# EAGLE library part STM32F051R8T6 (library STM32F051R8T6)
Entry-level ARM Cortex-M0 Access line MCU with 64 Kbytes Flash, 48 MHz CPU, motor control and CEC functions
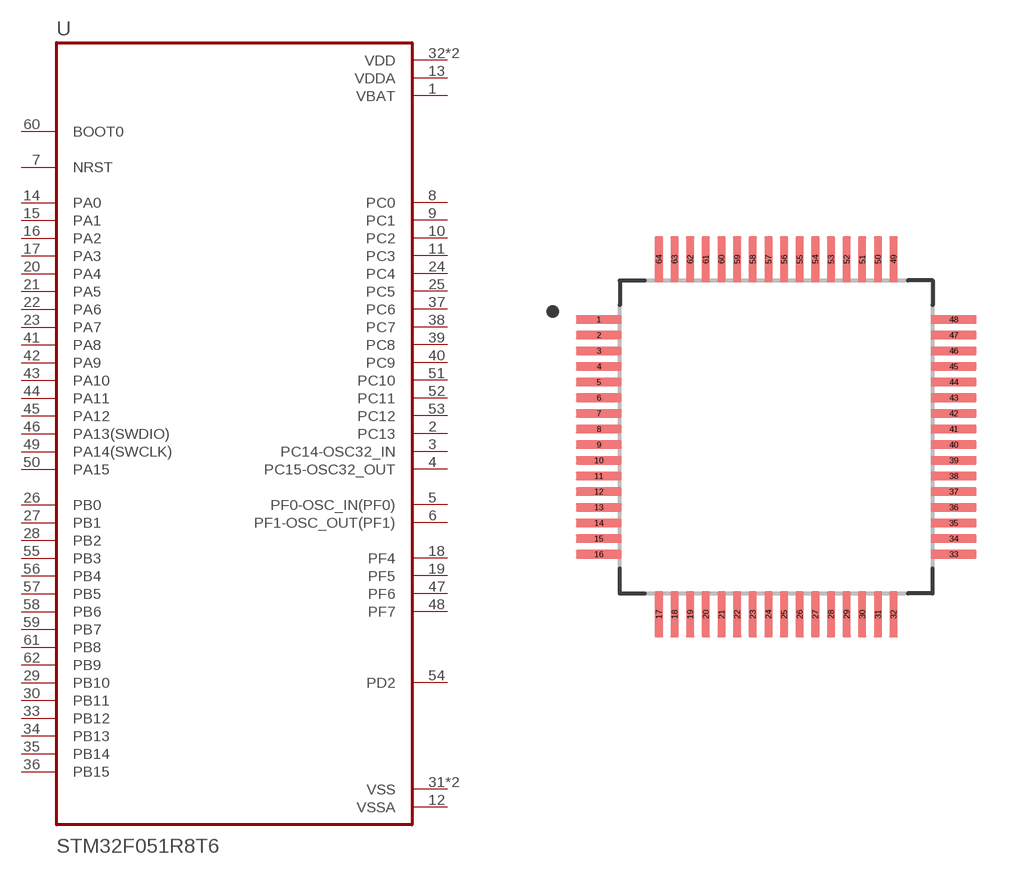
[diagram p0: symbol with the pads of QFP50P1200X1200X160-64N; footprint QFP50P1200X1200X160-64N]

Designator prefix U

## STM32F051R8T6 (AVAILABILITY: Unavailable; DESCRIPTION: Entry-level ARM Cortex-M0 MCU with 64 Kbytes Flash, 48 MHz CPU, motor control and CEC functions; MF: STMicroelectronics; MP: STM32F051R8T6; PACKAGE: LQFP-64 STMicroelectronics; PRICE: None)  [QFP50P1200X1200X160-64N]
1  VBAT  pwr
2  PC13
3  PC14-OSC32_IN
4  PC15-OSC32_OUT
5  PF0-OSC_IN(PF0)
6  PF1-OSC_OUT(PF1)
7  NRST
8  PC0
9  PC1
10  PC2
11  PC3
12  VSSA  pwr
13  VDDA  pwr
14  PA0
15  PA1
16  PA2
17  PA3
18  PF4
19  PF5
20  PA4
21  PA5
22  PA6
23  PA7
24  PC4
25  PC5
26  PB0
27  PB1
28  PB2
29  PB10
30  PB11
31  VSS  pwr
32  VDD  pwr
33  PB12
34  PB13
35  PB14
36  PB15
37  PC6
38  PC7
39  PC8
40  PC9
41  PA8
42  PA9
43  PA10
44  PA11
45  PA12
46  PA13(SWDIO)
47  PF6
48  PF7
49  PA14(SWCLK)
50  PA15
51  PC10
52  PC11
53  PC12
54  PD2
55  PB3
56  PB4
57  PB5
58  PB6
59  PB7
60  BOOT0  in
61  PB8
62  PB9
63  VSS  pwr
64  VDD  pwr

## Footprint QFP50P1200X1200X160-64N (pad centres in mm)
smd 1.47 x 0.28: 1 -5.67,3.75; 2 -5.67,3.25; 3 -5.67,2.75; 4 -5.67,2.25; 5 -5.67,1.75; 6 -5.67,1.25; 7 -5.67,0.75; 8 -5.67,0.25; 9 -5.67,-0.25; 10 -5.67,-0.75; 11 -5.67,-1.25; 12 -5.67,-1.75; 13 -5.67,-2.25; 14 -5.67,-2.75; 15 -5.67,-3.25; 16 -5.67,-3.75; 33 5.67,-3.75; 34 5.67,-3.25; 35 5.67,-2.75; 36 5.67,-2.25; 37 5.67,-1.75; 38 5.67,-1.25; 39 5.67,-0.75; 40 5.67,-0.25; 41 5.67,0.25; 42 5.67,0.75; 43 5.67,1.25; 44 5.67,1.75; 45 5.67,2.25; 46 5.67,2.75; 47 5.67,3.25; 48 5.67,3.75
smd 0.28 x 1.47: 17 -3.75,-5.67; 18 -3.25,-5.67; 19 -2.75,-5.67; 20 -2.25,-5.67; 21 -1.75,-5.67; 22 -1.25,-5.67; 23 -0.75,-5.67; 24 -0.25,-5.67; 25 0.25,-5.67; 26 0.75,-5.67; 27 1.25,-5.67; 28 1.75,-5.67; 29 2.25,-5.67; 30 2.75,-5.67; 31 3.25,-5.67; 32 3.75,-5.67; 49 3.75,5.67; 50 3.25,5.67; 51 2.75,5.67; 52 2.25,5.67; 53 1.75,5.67; 54 1.25,5.67; 55 0.75,5.67; 56 0.25,5.67; 57 -0.25,5.67; 58 -0.75,5.67; 59 -1.25,5.67; 60 -1.75,5.67; 61 -2.25,5.67; 62 -2.75,5.67; 63 -3.25,5.67; 64 -3.75,5.67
